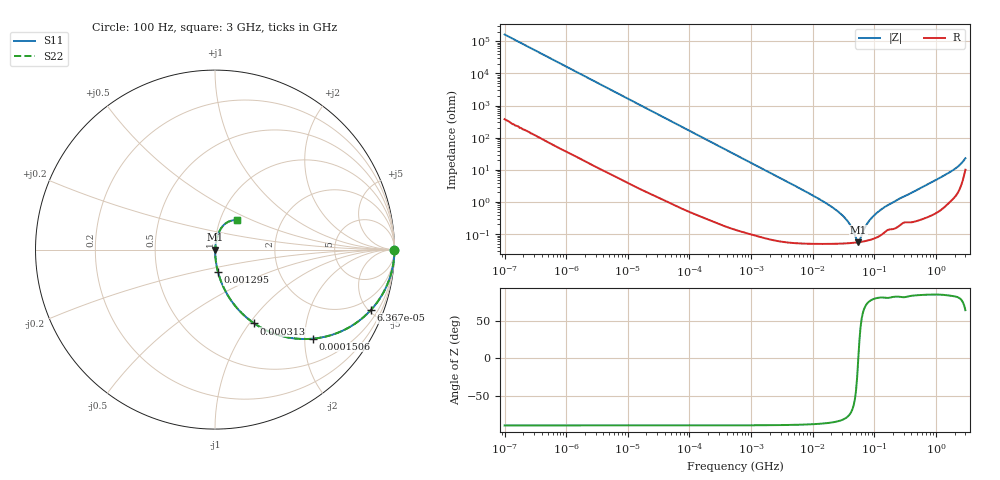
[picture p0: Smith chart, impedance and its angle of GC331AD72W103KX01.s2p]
!Murata Part Number: GC331AD72W103KX01
!These Parameters are Measured in Series Mode Connection
!Data Generated on Jan 08, 2026
!  o--ll--o
!Port1  Port2
!  o------o
!Operation Temp=25[degC], DC Bias Voltage=0[V]
!Freq. Start=100[Hz] Stop=3[GHz] 401[Steps]
# Hz S RI R 50
!Freq.(Hz) S11(Real) S11(Imag) S21(Real) S21(Imag) S12(Real) S12(Imag) S22(Real) S22(Imag)
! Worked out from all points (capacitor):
!   401 points, 100 Hz to 3 GHz, reference 50 ohm
!   read as one part in series: C = 9.76 nF near 109 Hz
!   lowest |Z| = 55.9 mohm at 54.79 MHz (marker M1)
!   series resonance near 54.92 MHz, so ESL is about 860 pH
!   S11 on the Smith chart (normalised r, x): 100 Hz: open; 63.67 kHz: 1.01, -5.17; 150.6 kHz: 1.01, -2.19; 313 kHz: 1.00, -1.05; 1.295 MHz: 1.00, -0.26; 3 GHz: 1.20, +0.41
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100  1 -0.000614  1.8e-06 0.000614  1.8e-06 0.000614  1 -0.000614
1788  0.9999 -0.0109  0.000144 0.0109  0.000144 0.0109  0.9999 -0.0109
10003  0.9962 -0.0607  0.00385 0.0607  0.00385 0.0607  0.9962 -0.0607
31977  0.9631 -0.1873  0.0369 0.1873  0.0369 0.1873  0.9631 -0.1873
63668  0.869 -0.336  0.131 0.336  0.131 0.336  0.869 -0.336
150583  0.5447 -0.4964  0.4553 0.4964  0.4553 0.4964  0.5447 -0.4964
313007  0.2183 -0.4112  0.7817 0.4112  0.7817 0.4112  0.2183 -0.4112
547723  0.0844 -0.2757  0.9156 0.2757  0.9156 0.2757  0.0844 -0.2757
1295438  0.0168 -0.1254  0.9832 0.1254  0.9832 0.1254  0.0168 -0.1254
9794414  0.000768 -0.0164  0.9992 0.0164  0.9992 0.0164  0.000768 -0.0164
1.950129e7  0.000553 -0.00742  0.9994 0.00742  0.9994 0.00742  0.000553 -0.00742
2.999103e7  0.000524 -0.00388  0.9995 0.00388  0.9995 0.00388  0.000524 -0.00388
3.882828e7  0.000528 -0.00213  0.9995 0.00213  0.9995 0.00213  0.000528 -0.00213
5.026954e7  0.000548 -0.000533  0.9995 0.000533  0.9995 0.000533  0.000548 -0.000533
5.478864e7  0.000559 -1.38e-05  0.9994 1.38e-05  0.9994 1.38e-05  0.000559 -1.38e-05
5.9714e7  0.000572 0.000506  0.9994 -0.000506  0.9994 -0.000506  0.000572 0.000506
7.093284e7  0.00061 0.00156  0.9994 -0.00156  0.9994 -0.00156  0.00061 0.00156
8.79653e7  0.000684 0.00294  0.9993 -0.00294  0.9993 -0.00294  0.000684 0.00294
1.241234e8  0.000925 0.00547  0.9991 -0.00547  0.9991 -0.00547  0.000925 0.00547
1.751444e8  0.00147 0.00829  0.9985 -0.00829  0.9985 -0.00829  0.00147 0.00829
1.573002e9  0.0147 0.0768  0.9853 -0.0768  0.9853 -0.0768  0.0147 0.0768
3e9  0.1224 0.1641  0.8776 -0.1641  0.8776 -0.1641  0.1224 0.1641
